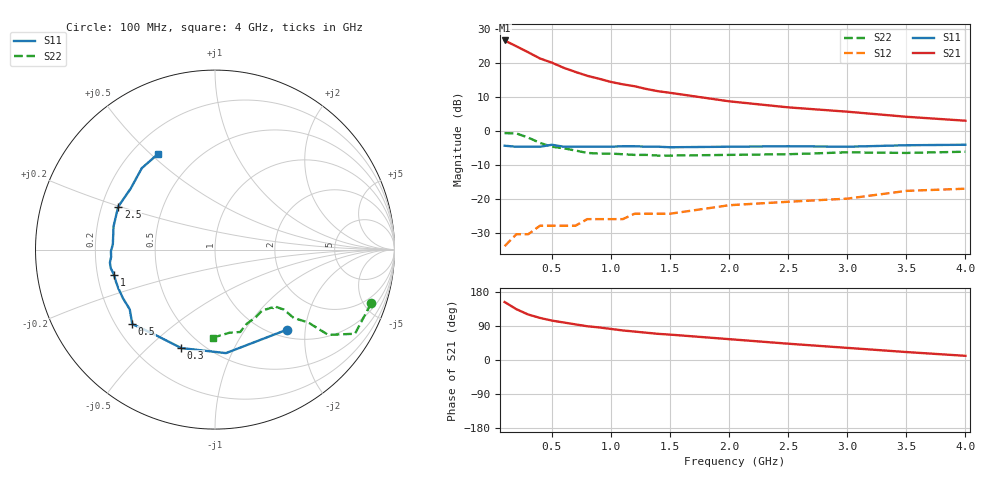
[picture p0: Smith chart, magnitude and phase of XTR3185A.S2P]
! HXTR-3185
! Typical S-Parameters  Vce =10 V, Ic = 10 mA
# ghz s ma r 50
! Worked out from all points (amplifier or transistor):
!   20 points, 100 MHz to 4 GHz, reference 50 ohm
!   highest |S21| = 26.5 dB at 100 MHz (marker M1)
!   |S21| within 3 dB of that: start of sweep to 272.8 MHz
!   unconditionally stable (mu >= 1): 1.338 GHz to end of sweep
!   at 400 MHz: K = 0.35, MSG = 24.6 dB, |S12| = -28.0 dB
!   at 1.1 GHz: K = 0.96, MSG = 19.8 dB, |S12| = -26.0 dB
!   at 4 GHz: K = 1.03, MAG = 9.0 dB, |S12| = -17.1 dB
!   S11 on the Smith chart (normalised r, x): 100 MHz: 1.15, -1.60; 300 MHz: 0.39, -0.64; 500 MHz: 0.27, -0.36; 1 GHz: 0.27, -0.11; 2.5 GHz: 0.27, +0.20; 4 GHz: 0.30, +0.53
0.1  0.6 -48.0  21.2 153.0  0.02 69.0  0.92 -19.0
0.2  0.58 -84.0  17.4 134.0  0.03 55.0  0.91 -31.0
0.3  0.58 -109.0  14.2 120.0  0.03 48.0  0.79 -37.0
0.4  0.58 -125.0  11.5 111.0  0.04 44.0  0.66 -38.0
0.5  0.62 -138.0  10 104.0  0.04 44.0  0.58 -41.0
0.6  0.58 -145.0  8.4 99.0  0.04 42.0  0.55 -41.0
0.7  0.58 -152.0  7.3 94.0  0.04 43.0  0.51 -41.0
0.8  0.58 -158.0  6.4 89.0  0.05 43.0  0.47 -43.0
0.9  0.58 -162.0  5.8 86.0  0.05 44.0  0.46 -43.0
1  0.58 -166.0  5.2 82.0  0.05 44.0  0.46 -45.0
1.1  0.59 -170.0  4.8 78.0  0.05 45.0  0.45 -46.0
1.2  0.59 -173.0  4.5 75.0  0.06 46.0  0.44 -49.0
1.3  0.58 -176.0  4.1 72.0  0.06 47.0  0.44 -49.0
1.4  0.58 -179.0  3.8 69.0  0.06 47.0  0.43 -51.0
1.5  0.57 177.0  3.6 67.0  0.06 48.0  0.43 -53.0
2  0.58 167.0  2.7 55.0  0.08 51.0  0.44 -59.0
2.5  0.59 156.0  2.2 43.0  0.09 52.0  0.45 -67.0
3  0.58 144.0  1.9 32.0  0.1 51.0  0.48 -73.0
3.5  0.61 132.0  1.6 21.0  0.13 50.0  0.47 -80.0
4  0.62 121.0  1.4 11.0  0.14 48.0  0.49 -91.0
